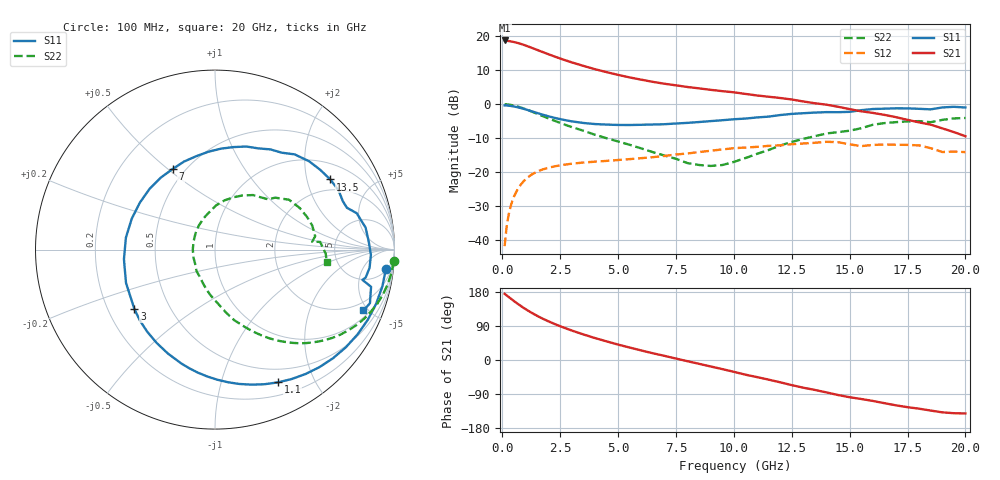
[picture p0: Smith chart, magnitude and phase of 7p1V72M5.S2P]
! Infineon Technologies  Discrete & RF Semiconductors
! bfp620
! VCE =  1.7 V,  IC =  2.5 mA
! Common Emitter S-Parameters:  Sep 2002
# GHz  S  MA  R  50
!  f  S11  S21  S12  S22
! GHz  MAG  ANG  MAG  ANG  MAG  ANG  MAG  ANG
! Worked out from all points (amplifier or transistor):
!   59 points, 100 MHz to 20 GHz, reference 50 ohm
!   highest |S21| = 18.7 dB at 100 MHz (marker M1)
!   |S21| within 3 dB of that: start of sweep to 1.59 GHz
!   unconditionally stable (mu >= 1): 5.564 GHz to 13.4 GHz; 14.22 GHz to 15.64 GHz; 17.44 GHz to end of sweep
!   at 1 GHz: K = 0.19, MSG = 19.7 dB, |S12| = -22.1 dB
!   at 5.5 GHz: K = 0.99, MSG = 12.0 dB, |S12| = -16.2 dB
!   at 20 GHz: K = 1.39, MAG = -1.4 dB, |S12| = -14.1 dB
!   S11 on the Smith chart (normalised r, x): 100 MHz: 6, -15; 1.1 GHz: 0.34, -1.53; 3 GHz: 0.31, -0.30; 7 GHz: 0.43, +0.52; 13.5 GHz: 1.55, +2.79; 20 GHz: 1.39, -4.68
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0.1  0.9581 -6.5  8.62 174.6  0.0082 83.6  0.9979 -3.8
0.3  0.9473 -18.6  8.42 165.2  0.0263 79.5  0.9822 -11.2
0.6  0.9096 -36.8  8.023 151.2  0.0513 69.4  0.935 -21.8
0.8  0.876 -48.4  7.675 142.6  0.0658 62.7  0.8922 -28.2
1.1  0.8188 -64.6  7.073 130.7  0.084 53.5  0.8197 -36.8
1.3  0.7798 -74.8  6.662 123.5  0.0938 48.2  0.7702 -41.7
1.5  0.7426 -84.4  6.271 116.7  0.1018 43.4  0.7224 -46.2
2  0.6624 -106.3  5.401 101.9  0.1164 33.8  0.6171 -55.3
2.4  0.613 -122.1  4.811 91.5  0.1246 27.8  0.5466 -61.3
3  0.5583 -143.5  4.109 77.8  0.1332 20.6  0.4611 -69.0
3.5  0.5294 -159.5  3.65 67.5  0.1389 15.7  0.4072 -74.8
4  0.5101 -174.0  3.264 58.0  0.1428 11.6  0.3554 -80.1
5  0.4948 159.6  2.691 40.7  0.1512 5.6  0.2833 -89.9
6  0.4975 137.1  2.289 25.2  0.1609 0.4  0.2239 -102.9
7  0.5071 117.8  1.994 11.0  0.1733 -4.2  0.1759 -118.3
8.5  0.5464 93.9  1.705 -10.1  0.1978 -12.9  0.1277 -160.3
10.5  0.6138 66.7  1.413 -38.7  0.2305 -29.2  0.1614 124.1
12  0.6916 50.1  1.232 -58.8  0.2485 -40.8  0.2464 88.6
13.5  0.7519 31.3  1.031 -79.0  0.2707 -54.8  0.3385 63.0
15  0.7709 17.6  0.845 -98.2  0.2571 -74.3  0.4071 43.5
17  0.8692 -1.9  0.644 -119.6  0.2533 -86.0  0.544 19.6
20  0.8936 -22.3  0.338 -141.1  0.1976 -105.4  0.6262 -6.2
